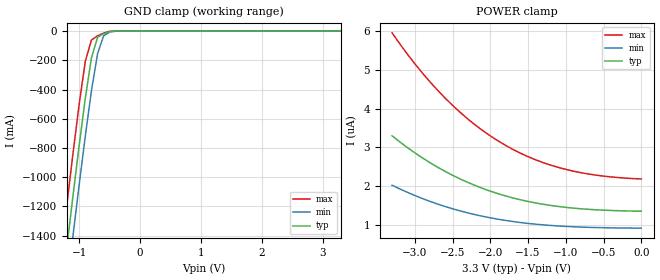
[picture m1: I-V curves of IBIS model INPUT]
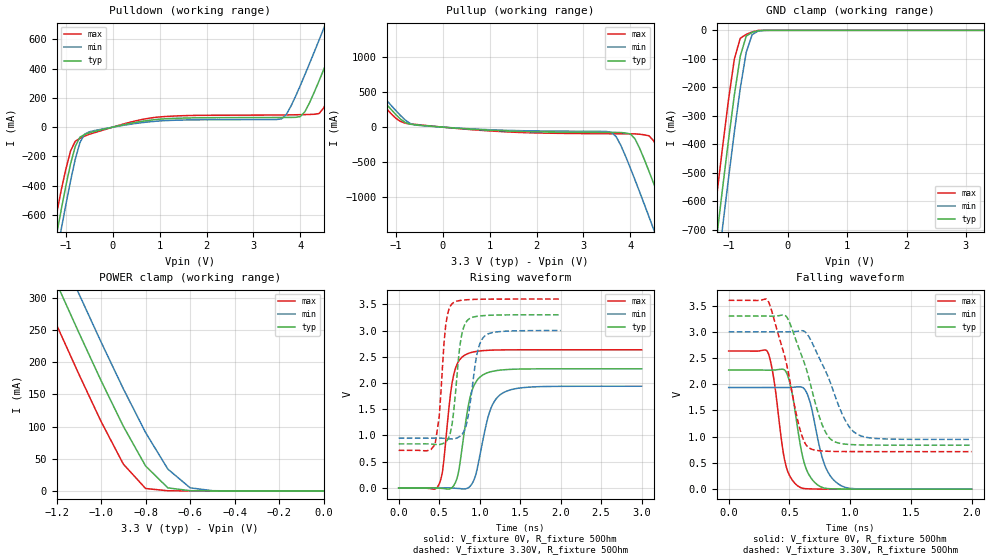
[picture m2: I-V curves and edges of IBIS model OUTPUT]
|   PERICOM SEMICONDUCTOR CORP
|   IBIS Model of PI90LV02
|   Product Family: 90LV
|   SOT23 Package (T)
[IBIS Ver] 3.2
[Comment char] |_char
[File Name] pi90lv02_t_reva.ibs
[File Rev] 1.0
[Source] File originated at Pericom Semiconductor Corp.
[Date] 10/16/17
[Disclaimer] (C) Copyright PERICOM Semiconductor Corporation
   All rights reserved
  Pericom Semiconductor Corporation hereby grants the user of
  this IBIS model a non-exclusive, nontransferable license to
  use this IBIS model under the following terms.
  This IBIS model is provided on an "AS IS" basis and Pericom
  makes absolutely no warranty with respect to the information
  contained herein. PERICOM DISCLAIMS AND CUSTOMER WAIVES ALL
  WARRANTIES, EXPRESSED OR IMPLIED, INCLUDING WARRANTIES OF
  MERCHANTABILITY OR FITNESS FOR A PARTICULAR PURPOSE. The
  entire risk as to quality and performance is with the customer.
  Accordingly, in no event shall the company be liable for any
  damages, whether in contract or tort, including any lost
  profits or other incidental, consequential, exemplary, or
  punitive damages arising out of the use or application of the
  IBIS model provided in this package. Further, Pericom reserves
  the right to make changes without notice to any product herein
  to improve reliability, function, or design. Pericom does not
  convey any license under patent rights or any other intellectual
  property rights, including those of third parties.
  The user is granted this license only to use the IBIS model
  and is not granted rights to sell, load, rent, lease or license
  the IBIS model in whole or in part, or in modified form to anyone
  other than user. User may modify the IBIS model to suit its specific
  application but rights to derivative works and such modifications
  shall belong to Pericom.
  Pericom is not obligated to provide maintenance or support
  for the licensed IBIS model.
  Contact Pericom at ATTN: APPLICATIONS ENGINEERING / IBIS MODELS
  1545 Barber Lane Milpitas, CA 95035 USA.
[Component] PI90LV02
[Manufacturer] Pericom Semiconductor Corp.
[Package]
| variable   typ   min   max
R_pkg   0.06523ohm   0.05910ohm   0.07136ohm
L_pkg   3.84667nH   3.49400nH   4.19933nH
C_pkg   0.49367pF   0.47000pF   0.51733pF
[Pin]  signal_name   model_name   R_pin   L_pin   C_pin
1   VCC   POWER   0.05660   3.27800nH   0.43000pF
2   GND   GND   0.04020   2.86800nH   0.38000pF
3   A   INPUT   0.05660   3.27800nH   0.43000pF
4   B   INPUT   0.05660   3.27800nH   0.43000pF
5   ROUT   OUTPUT   0.05660   3.27800nH   0.43000pF
[Diff Pin] inv_pin vdiff  tdelay_typ tdelay_min tdelay_max
4   3   350mv  NA   NA   NA
| Models and submodels in the file (2): INPUT (Input), OUTPUT (Output)
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|   Model INPUT
[Model] INPUT
Model_type Input
Vinl = 800mV
Vinh = 2.00V
| variable   typ   min   max
C_comp   2.50p   2.45p   2.55p
[Voltage Range]   3.30V   3.00V   3.60V
[POWER Clamp Reference]   3.30V   3.00V   3.60V
[GND Clamp Reference]   0.00V   0.00V   0.00V
[temperature range]   25   85   -40
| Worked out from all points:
|   GND clamp passes 1 mA (typ) near -0.42 V on its own axis
[GND Clamp]
| Voltage   I(typ)   I(min)   I(max)
-3.3V     -9.197A    -9.452A    -8.929A
-1.3V     -1.822A    -2.095A    -1.532A
-1.2V     -1.467A    -1.74A     -1.176A
-1.1V     -1.118A    -1.39A     -828.5mA
-1V       -777.9mA   -1.047A    -495.9mA
-900mV    -457mA     -716.5mA   -205.6mA
-800mV    -183.8mA   -408.8mA   -61.31mA
-700mV    -44.07mA   -156.5mA   -32.71mA
-600mV    -16.67mA   -32.34mA   -13.48mA
-500mV    -3.475mA   -6.341mA   -1.316mA
-400mV    -273.6uA   -967.8uA   -24.93uA
3.3V      1.359uA    927.6nA    2.172uA
[POWER Clamp]
| Voltage   I(typ)   I(min)   I(max)
-3.3V     3.3uA      2.028uA    5.95uA
-3V       2.864uA    1.764uA    5.158uA
-2.8V     2.611uA    1.613uA    4.693uA
-2.6V     2.387uA    1.481uA    4.276uA
-2.4V     2.19uA     1.367uA    3.906uA
-2.2V     2.021uA    1.27uA     3.581uA
-2V       1.876uA    1.189uA    3.299uA
-1.8V     1.754uA    1.122uA    3.057uA
-1.4V     1.572uA    1.025uA    2.683uA
-1V       1.459uA    967.8nA    2.436uA
-500mV    1.386uA    933.9nA    2.263uA
0V        1.359uA    922.5nA    2.189uA
|   Model OUTPUT
[Model]   OUTPUT
Model_type  Output
Vref =  1.650V
Vmeas = 1.650V
| variable   typ   min   max
C_comp   2.50p   2.45p   2.55p
[Voltage Range]   3.30V   3.00V   3.60V
[Temperature Range]   25   85   -40
[Pullup Reference]   3.30V   3.00V   3.60V
[Pulldown Reference]   0.00V   0.00V   0.00V
[POWER Clamp Reference]   3.30V   3.00V   3.60V
[GND Clamp Reference]   0.00V   0.00V   0.00V
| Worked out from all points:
|   slope of the pulldown table from 0 to 0.495 V, typ, clamps not added: 15 ohm
|   slope of the pullup table from 0 to 0.495 V, typ, clamps not added: 20.3 ohm
|   GND clamp passes 1 mA (typ) near -0.47 V on its own axis
|   POWER clamp passes 1 mA (typ) near -0.61 V on its own axis
|   falling waveform, V_fixture 0V, R_fixture 50Ohm: 20-80 % time 105ps typ, 122ps min, 92.3ps max; typ from 2.27 V to 0 V
|   rising waveform, V_fixture 0V, R_fixture 50Ohm: 20-80 % time 143ps typ, 176ps min, 115ps max; typ from 0 V to 2.27 V
|   falling waveform, V_fixture 3.30V, R_fixture 50Ohm: 20-80 % time 194ps typ, 222ps min, 171ps max; typ from 3.3 V to 0.839 V
|   rising waveform, V_fixture 3.30V, R_fixture 50Ohm: 20-80 % time 96.7ps typ, 116ps min, 81.1ps max; typ from 0.839 V to 3.3 V
[GND Clamp]
| Voltage   I(typ)   I(min)   I(max)
-3.3V     -4.59A     -4.717A    -4.456A
-1.3V     -908.8mA   -1.045A    -763.8mA
-1.2V     -731.6mA   -868.1mA   -586.3mA
-1.1V     -557.2mA   -693.4mA   -412.5mA
-1V       -387.5mA   -522.2mA   -246.3mA
-900mV    -227.2mA   -357mA     -100.8mA
-800mV    -90.44mA   -203.3mA   -27.66mA
-700mV    -20.23mA   -77.17mA   -14.17mA
-600mV    -7.162mA   -15.09mA   -5.633mA
-500mV    -1.35mA    -2.642mA   -477uA
-400mV    -96.44uA   -360.5uA   -7.402uA
3.3V      172.6pA    2.118uA    57.7pA
[POWER Clamp]
| Voltage   I(typ)   I(min)   I(max)
-3.3V     2.018A     2.074A     1.958A
-1.3V     401.1mA    461.6mA    336.6mA
-1.2V     323.1mA    383.8mA    258.5mA
-1.1V     246.4mA    307mA      181.8mA
-1V       171.6mA    231.7mA    108mA
-900mV    100.6mA    158.8mA    41.73mA
-800mV    38.75mA    90.75mA    3.781mA
-700mV    4.724mA    33.91mA    245.8uA
-600mV    359.8uA    4.823mA    23.01uA
-500mV    28.11uA    369.6uA    585.2nA
0V        172.6pA    6.113nA    72.13pA
[Pulldown]
| Voltage   I(typ)   I(min)   I(max)
-3.3V     -4.591A    -4.718A    -4.457A
-1.3V     -912.9mA   -1.048A    -770mA
-1.1V     -564.5mA   -697.7mA   -430.3mA
-800mV    -131.4mA   -218.6mA   -96.08mA
-600mV    -50.61mA   -47.96mA   -61.43mA
900mV     51.39mA    39.78mA    66.4mA
3.6V      66.04mA    56.75mA    83.19mA
4V        71.88mA    284.4mA    85.04mA
4.4V      316mA      594.6mA    92.75mA
4.9V      714.9mA    997.8mA    435.1mA
5.2V      961.9mA    1.244A     682.5mA
6.6V      2.159A     2.429A     1.897A
[Pullup]
| Voltage   I(typ)   I(min)   I(max)
-3.3V     2.018A     2.075A     1.959A
-2.7V     1.529A     1.586A     1.468A
-2.5V     1.366A     1.424A     1.305A
-1.2V     326.9mA    386.5mA    264.1mA
-800mV    66.07mA    101.5mA    55.73mA
3.6V      -75.58mA   -75.74mA   -94.55mA
4V        -96.72mA   -583.6mA   -95.65mA
4.4V      -634.5mA   -1.286A    -124.3mA
4.5V      -809.1mA   -1.466A    -197.6mA
4.8V      -1.346A    -2.012A    -683.8mA
5.2V      -2.077A    -2.746A    -1.405A
6.6V      -4.672A    -5.341A    -3.999A
[Falling Waveform]
V_fixture = 0V
V_fixture_min = 0V
V_fixture_max = 0V
R_fixture = 50Ohm
C_fixture = 0F
|   Time   V(typ)   V(min)   V(max)
0s        2.27V      1.938V     2.633V
320ps     2.269V     1.938V     2.622V
370ps     2.27V      1.938V     2.125V
480ps     2.2V       1.937V     378.4mV
580ps     976.7mV    1.951V     45.58mV
630ps     440.7mV    1.89V      10.37mV
690ps     174.8mV    1.467V     4.163mV
790ps     19.11mV    463.4mV    1.202mV
920ps     2.929mV    73.5mV     270.3uV
2ns       0V         1.602uV    0V
[Rising Waveform]
V_fixture = 0V
V_fixture_min = 0V
V_fixture_max = 0V
R_fixture = 50Ohm
C_fixture = 0F
|   Time   V(typ)   V(min)   V(max)
0s        -25.47uV   -8.788uV   66.61uV
500ps     -5.2mV     566.9uV    72.38mV
540ps     -10.05mV   958.9uV    295.8mV
660ps     6.183mV    -3.013mV   2.006V
730ps     238.1mV    -10.13mV   2.387V
810ps     1.064V     -20.46mV   2.525V
960ps     2.035V     298.4mV    2.603V
1.12ns    2.207V     1.437V     2.624V
1.3ns     2.252V     1.821V     2.631V
3ns       2.27V      1.938V     2.633V
[Falling Waveform]
V_fixture = 3.30V
V_fixture_min = 3.00V
V_fixture_max = 3.60V
R_fixture = 50Ohm
C_fixture = 0F
|   Time   V(typ)   V(min)   V(max)
0s        3.3V       3V         3.6V
330ps     3.299V     3V         3.564V
480ps     3.275V     2.998V     2.348V
580ps     2.674V     3.015V     1.2V
660ps     2.12V      2.909V     789.7mV
750ps     1.355V     2.48V      731.8mV
820ps     1.002V     2.137V     722.1mV
960ps     859.1mV    1.31V      716.9mV
1.06ns    845mV      1.044V     716.1mV
2ns       838.7mV    948.7mV    715.8mV
[Rising Waveform]
V_fixture = 3.30V
V_fixture_min = 3.00V
V_fixture_max = 3.60V
R_fixture = 50Ohm
C_fixture = 0F
|   Time   V(typ)   V(min)   V(max)
0s        838.8mV    948.7mV    715.9mV
450ps     829.3mV    949.5mV    831.7mV
500ps     826.5mV    948.8mV    1.346V
580ps     875.8mV    942.9mV    3.088V
660ps     1.217V     933.1mV    3.512V
760ps     2.75V      987.3mV    3.574V
850ps     3.195V     1.302V     3.588V
960ps     3.269V     2.495V     3.595V
1.05ns    3.284V     2.876V     3.598V
2ns       3.3V       3V         3.6V
[Ramp]
| variable   typ   min   max
dV/dt_r   1.36224V/142.47p   1.16274V/178.82p   1.57992V/115.02p
dV/dt_f   1.47678V/194.54p   1.23078V/221.93p   1.73052V/170.51p
